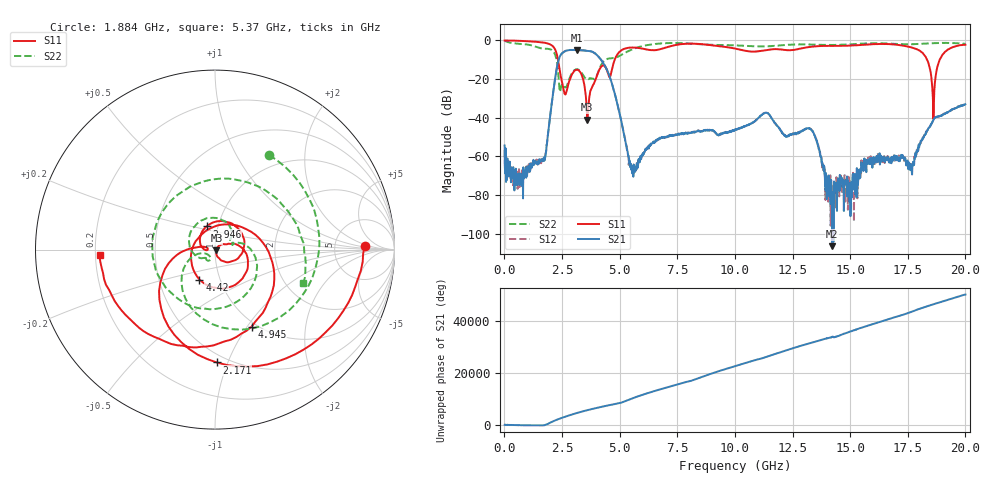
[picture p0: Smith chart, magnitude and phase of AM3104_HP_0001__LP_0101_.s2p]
!Created with skrf (http://scikit-rf.org).
# Hz S RI R 50.0
!freq ReS11 ImS11 ReS21 ImS21 ReS12 ImS12 ReS22 ImS22
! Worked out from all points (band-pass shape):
!   1601 points, 10 MHz to 20 GHz, reference 50 ohm
!   highest |S21| = -4.86 dB at 3.133 GHz (marker M1); lowest = -106.5 dB at 14.23 GHz (marker M2)
!   |S21| within 3 dB of the highest: 2.425 GHz to 4.044 GHz (1.619 GHz wide, 50.1 % of centre)
!   lowest |S11| = -41.0 dB at 3.596 GHz (marker M3), VSWR 1.02, Z = 50.8 - j0.456 ohm
!   |S11| at or under -10 dB: 2.326 GHz to 4.786 GHz (2.46 GHz wide, 69.2 % of centre); 18.34 GHz to 18.88 GHz (543.9 MHz wide, 2.92 % of centre)
!   |S22| runs from -26.6 to -0.2 dB; largest |S21 - S12| = 0.0063
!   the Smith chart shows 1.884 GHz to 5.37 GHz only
!   S11 on the Smith chart (normalised r, x): 1.884 GHz: 11, +2; 2.171 GHz: 0.44, -0.91; 2.946 GHz: 0.88, +0.23; 4.42 GHz: 0.80, -0.28; 4.945 GHz: 0.94, -1.05; 5.37 GHz: 0.22, -0.02
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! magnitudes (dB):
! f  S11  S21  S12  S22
! 10 MHz  0.0  -54.4  -56.7  -0.2
! 709.6 MHz  -0.2  -69.9  -69.9  -1.8
! 1.884 GHz  -1.6  -49.2  -49.3  -4.3
! 2.171 GHz  -4.0  -22.2  -22.2  -6.6
! 2.609 GHz  -27.5  -5.7  -5.7  -24.0
! 2.946 GHz  -17.2  -4.9  -4.9  -16.6
! 3.133 GHz  -15.2  -4.9  -4.9  -14.9
! 3.346 GHz  -17.6  -5.1  -5.1  -16.6
! 3.596 GHz  -41.0  -5.4  -5.4  -20.1
! 4.42 GHz  -14.5  -14.4  -14.4  -9.8
! 4.945 GHz  -6.5  -35.0  -35.0  -8.3
! 5.37 GHz  -3.8  -59.6  -59.5  -5.6
! 5.632 GHz  -3.7  -64.9  -64.8  -4.2
! 6.682 GHz  -4.7  -50.8  -51.3  -1.7
! 10.01 GHz  -4.2  -46.5  -46.4  -2.5
! 13.34 GHz  -3.2  -46.6  -46.4  -2.2
! 14.23 GHz  -2.8  -106.5  -87.2  -2.3
! 16.68 GHz  -1.9  -60.9  -62.2  -1.6
! 17.69 GHz  -3.7  -69.4  -64.2  -1.9
! 18.61 GHz  -40.7  -41.2  -41.1  -1.4
! 19.01 GHz  -7.3  -38.4  -38.4  -1.3
! 20 GHz  -2.2  -33.0  -33.0  -1.7
